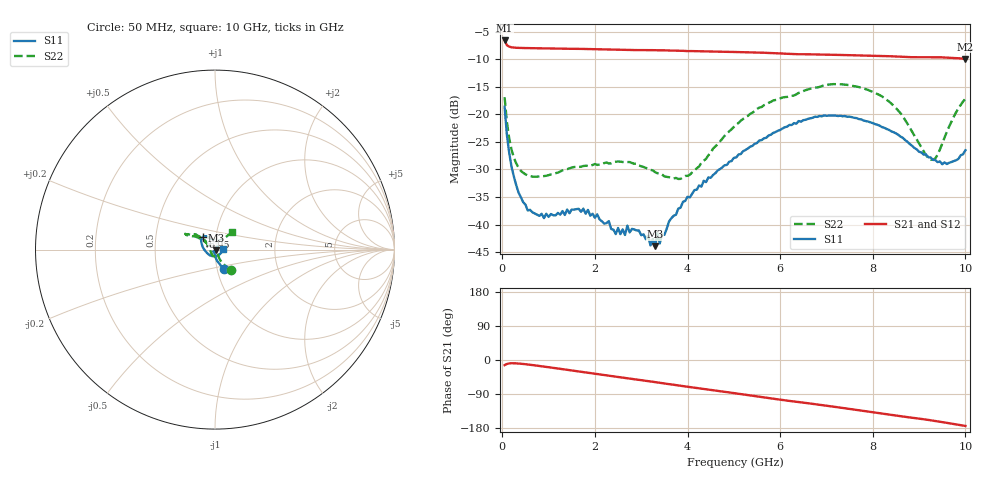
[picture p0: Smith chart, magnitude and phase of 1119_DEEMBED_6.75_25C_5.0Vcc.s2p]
!Hittite Microwave Corp.
!Digital Attenuator/PhaseShifter Rev 1.4.0
!Filename: C:\DATA\DATA\1119_DEEMBED_6.75_25C_5.0Vcc.s2p
!VNA ID: Agilent Technologies,N5224A,MY51441122,A.10.45.03
!Device type:
!2 Port Calibration.
!Temp(C): 25
!Lot Number:
!Serial Number:
!Operator:
!Misc:
!Attenuator:  6.750
# GHZ S DB R 50.0
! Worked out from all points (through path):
!   200 points, 50 MHz to 10 GHz, reference 50 ohm
!   highest |S21| = -6.61 dB at 50 MHz (marker M1); lowest = -9.9 dB at 10 GHz (marker M2)
!   group delay of S21, straight-line fit = 46.9 ps
!   lowest |S11| = -43.9 dB at 3.3 GHz (marker M3), VSWR 1.01, Z = 50.6 - j0.313 ohm
!   |S11| at or under -10 dB: start of sweep to end of sweep
!   |S22| runs from -31.7 to -14.5 dB; largest |S21 - S12| = 0.0013
!   S11 on the Smith chart (normalised r, x): 50 MHz: 1.07, -0.23; 6.95 GHz: 0.87, +0.13; 10 GHz: 1.10, +0.00
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0.05  -18.65 -66.0  -6.61 -13.5  -6.61 -13.5  -16.91 -52.4
0.15  -27.04 -85.9  -7.74 -9.0  -7.74 -9.0  -24.42 -64.0
0.25  -31.30 -93.6  -7.90 -8.5  -7.91 -8.5  -27.88 -62.7
0.55  -37.46 -109.5  -8.00 -11.8  -8.00 -11.8  -31.10 -58.1
0.9  -38.84 -119.0  -8.05 -17.4  -8.05 -17.4  -31.22 -61.8
1.75  -37.13 -122.2  -8.15 -31.9  -8.15 -31.9  -29.38 -78.7
2.3  -39.39 -113.6  -8.24 -41.5  -8.24 -41.5  -28.93 -93.4
2.45  -41.74 -99.8  -8.29 -44.0  -8.30 -44.1  -28.62 -97.3
2.65  -41.90 -86.8  -8.34 -47.4  -8.34 -47.5  -28.64 -104.1
2.7  -40.21 -78.0  -8.34 -48.1  -8.34 -48.2  -28.67 -105.0
3.3  -43.93 -29.1  -8.39 -58.4  -8.40 -58.4  -30.50 -129.1
3.35  -41.57 -16.4  -8.39 -59.2  -8.41 -59.3  -30.70 -130.5
3.4  -43.44 -16.9  -8.39 -60.0  -8.40 -60.1  -30.74 -133.0
3.6  -39.45 11.9  -8.44 -63.7  -8.45 -63.8  -31.41 -142.4
4.05  -35.08 31.9  -8.53 -71.3  -8.54 -71.3  -30.98 -179.2
5.05  -27.85 81.0  -8.71 -88.2  -8.73 -88.2  -21.92 137.1
6.7  -20.64 128.2  -9.14 -115.8  -9.16 -115.8  -15.26 150.1
6.95  -20.20 132.5  -9.19 -119.8  -9.20 -119.8  -14.74 152.0
8.35  -22.84 164.9  -9.47 -143.9  -9.47 -143.9  -17.69 146.4
9.3  -28.28 -112.0  -9.64 -160.0  -9.66 -160.0  -28.26 104.0
9.6  -29.02 -65.0  -9.72 -165.9  -9.73 -165.9  -23.17 55.4
10  -26.54 1.5  -9.95 -174.0  -9.95 -174.0  -17.20 45.6
